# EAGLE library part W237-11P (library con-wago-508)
WAGO SREW CLAMP
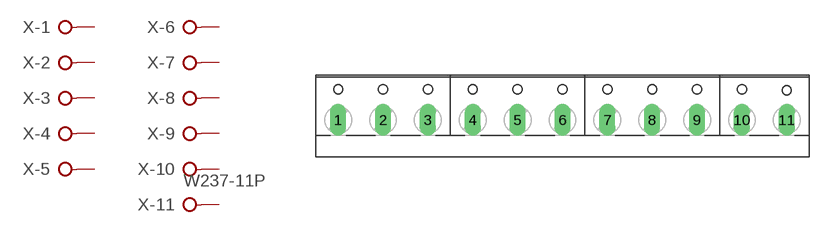
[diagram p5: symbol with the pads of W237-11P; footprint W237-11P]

Designator prefix X; gates -1=KL -2=KL -3=KL -4=KL -5=KL -6=KL -7=KL -8=KL -9=KL -10=KL -11=KL+V

## W237-11P (OC_FARNELL: unknown; OC_NEWARK: unknown)  [W237-11P]
1  -1:KL  pas
2  -2:KL  pas
3  -3:KL  pas
4  -4:KL  pas
5  -5:KL  pas
6  -6:KL  pas
7  -7:KL  pas
8  -8:KL  pas
9  -9:KL  pas
10  -10:KL  pas
11  -11:KL  pas

## Footprint W237-11P (pad centres in mm)
WAGO SREW CLAMP
drill 1.194 long: 1 -25.4,-0.635; 2 -20.32,-0.635; 3 -15.24,-0.635; 4 -10.16,-0.635; 5 -5.08,-0.635; 6 0,-0.635; 7 5.08,-0.635; 8 10.16,-0.635; 9 15.24,-0.635; 10 20.32,-0.635; 11 25.4,-0.635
